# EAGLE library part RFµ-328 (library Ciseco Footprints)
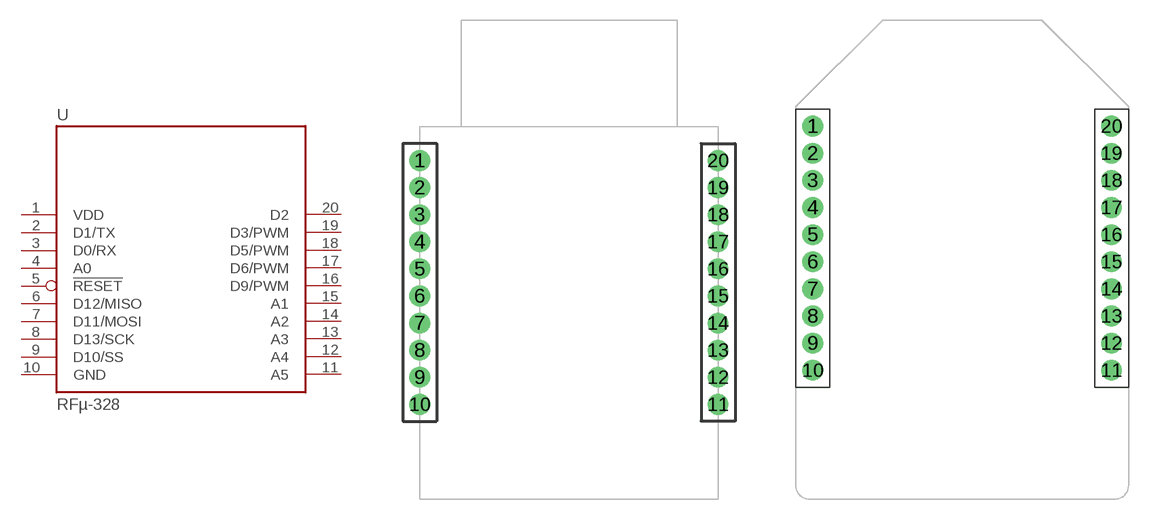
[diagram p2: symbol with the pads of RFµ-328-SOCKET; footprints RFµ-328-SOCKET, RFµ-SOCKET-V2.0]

Designator prefix U

## RFµ-328-SOCKET  [RFµ-328-SOCKET]
1  VDD  pwr
2  D1/TX  out
3  D0/RX  in
4  A0
5  !RESET  in
6  D12/MISO
7  D11/MOSI
8  D13/SCK
9  D10/SS
10  GND  pwr
11  A5
12  A4  out
13  A3
14  A2
15  A1
16  D9/PWM  in
17  D6/PWM
18  D5/PWM
19  D3/PWM
20  D2

## RFµ-328-SOCKET-V2.0  [RFµ-SOCKET-V2.0]
Pads as for RFµ-328-SOCKET

## RFµ-328-SOCKET-SMD-V2.0  [RFµ-SOCKET-SMD-V2.0]
Pads as for RFµ-328-SOCKET

## Footprint RFµ-328-SOCKET (pad centres in mm)
drill 0.8 pad 1.524: 1 -11,20; 2 -11,18; 3 -11,16; 4 -11,14; 5 -11,12; 6 -11,10; 7 -11,8; 8 -11,6; 9 -11,4; 10 -11,2; 11 11,2; 12 11,4; 13 11,6; 14 11,8; 15 11,10; 16 11,12; 17 11,14; 18 11,16; 19 11,18; 20 11,20

## Footprint RFµ-SOCKET-V2.0 (pad centres in mm)
drill 0.8 pad 1.524: 1 -11,20; 2 -11,18; 3 -11,16; 4 -11,14; 5 -11,12; 6 -11,10; 7 -11,8; 8 -11,6; 9 -11,4; 10 -11,2; 11 11,2; 12 11,4; 13 11,6; 14 11,8; 15 11,10; 16 11,12; 17 11,14; 18 11,16; 19 11,18; 20 11,20

## Footprint RFµ-SOCKET-SMD-V2.0 (pad centres in mm)
smd 1.7 x 0.85: 1 -12.5,20; 2 -9.5,18; 3 -12.5,16; 4 -9.5,14; 5 -12.5,12; 6 -9.5,10; 7 -12.5,8; 8 -9.5,6; 9 -12.5,4; 10 -9.5,2; 11 12.5,2; 12 9.5,4; 13 12.5,6; 14 9.5,8; 15 12.5,10; 16 9.5,12; 17 12.5,14; 18 9.5,16; 19 12.5,18; 20 9.5,20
